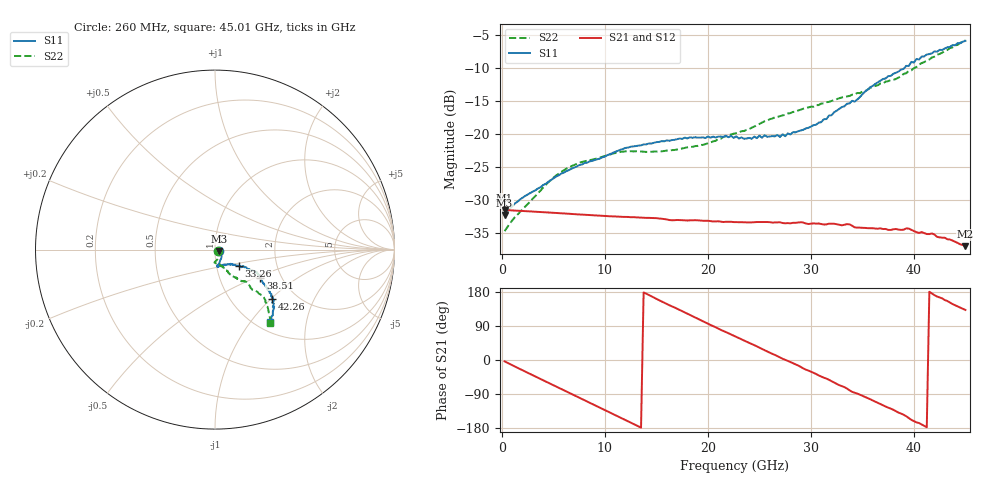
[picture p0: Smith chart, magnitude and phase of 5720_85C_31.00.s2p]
! Device:  ADRF5720
! Description: 0.5dB LSB GaAs MMIC 6-bit Digital Attenuator
! Frequency:  0.000009 -  40 GHz
! Ports:
!	RF1	= Port 1
!	RF2	= Port 2
! Vdd:  3.3 Volt
! Vss:  -3.3 Volt
! Control:  0/3.3 Volt
! State:  31.00 dB attenuation
! Data:  The device was measured using G-S-G Probes on a matrix board.
!  Data was collected using an calibrated 4 port network analyzer.
!  The reference plane for this measurement is at the launchers.
! Note:  Analog Devices supplies this data as a sample of measured data
!  for this product.  Your particular data for this product may vary.
!  Data was taken at 85 degrees C.
!  Analog Devices reserves the right to change this data at anytime.
# GHZ S DB R 45.0
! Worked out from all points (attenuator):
!   180 points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, 260 MHz to 45.01 GHz, reference 45 ohm
!   highest |S21| = -31.53 dB at 260 MHz (marker M1); lowest = -37.0 dB at 45.01 GHz (marker M2)
!   lowest |S11| = -32.3 dB at 260 MHz (marker M3), VSWR 1.05, Z = 47.1 - j0.736 ohm
!   |S11| at or under -10 dB: start of sweep to 39.08 GHz
!   |S22| runs from -34.7 to -5.8 dB; largest |S21 - S12| = 0.0002
!   S11 on the Smith chart (normalised r, x): 260 MHz: 1.05, -0.02; 33.26 GHz: 1.28, -0.24; 38.51 GHz: 1.57, -0.53; 42.26 GHz: 1.51, -1.02; 45.01 GHz: 1.15, -1.26
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0.26  -32.28 -18.7  -31.53 -3.7  -31.53 -3.7  -34.73 -26.4
1.76  -29.93 -5.0  -31.66 -23.9  -31.65 -23.9  -31.81 -20.6
4.76  -27.00 -36.9  -31.93 -63.5  -31.92 -63.4  -26.95 -65.7
6.26  -25.62 -46.2  -32.07 -83.0  -32.06 -83.0  -25.26 -75.2
7.76  -24.64 -53.8  -32.22 -102.6  -32.20 -102.5  -24.26 -81.6
11.51  -22.39 -70.1  -32.55 -151.7  -32.54 -151.7  -22.72 -92.1
15.26  -21.21 -78.7  -32.82 157.8  -32.80 158.0  -22.63 -89.9
19.51  -20.51 -82.0  -33.16 102.4  -33.15 102.6  -21.66 -76.5
22.76  -20.36 -77.7  -33.36 60.7  -33.34 60.9  -19.87 -67.3
24.26  -20.73 -74.3  -33.40 42.2  -33.39 42.4  -19.04 -64.4
25.01  -20.26 -71.6  -33.35 32.5  -33.33 32.7  -18.47 -64.2
27.51  -20.34 -60.6  -33.54 0.6  -33.52 0.9  -17.11 -59.4
30.26  -18.66 -45.6  -33.55 -33.9  -33.53 -33.6  -15.87 -58.5
33.26  -15.81 -34.1  -33.76 -71.6  -33.74 -71.3  -14.39 -53.8
37.76  -11.19 -29.5  -34.55 -128.4  -34.52 -128.0  -11.81 -46.1
38.51  -10.54 -31.6  -34.49 -138.8  -34.47 -138.4  -11.45 -45.9
39.51  -9.69 -34.6  -34.34 -153.3  -34.32 -152.9  -10.43 -46.9
40.26  -8.63 -36.9  -34.88 -164.5  -34.87 -164.2  -9.84 -45.4
41.76  -7.77 -39.8  -35.08 175.7  -35.05 176.1  -8.40 -44.3
42.26  -7.53 -41.2  -35.60 167.4  -35.54 167.8  -7.98 -45.2
43.51  -6.79 -43.9  -36.00 151.8  -36.00 152.2  -6.97 -48.6
45.01  -5.88 -53.0  -37.01 132.1  -37.02 132.4  -5.82 -53.3
